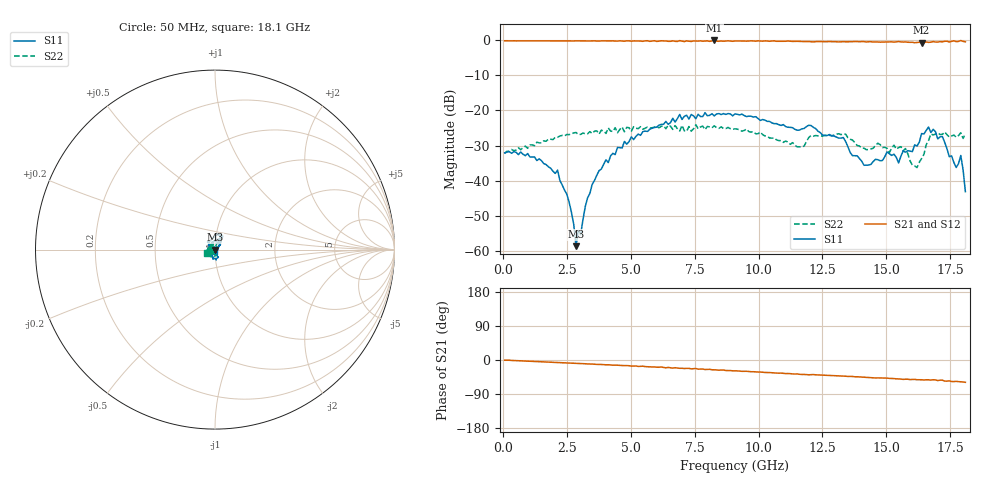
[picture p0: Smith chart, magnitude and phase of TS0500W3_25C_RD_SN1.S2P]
! Network Analyzer HP8720D.06.14 Serial No. US36140669
! 17 Jun 2005  06:18:02
! Frequency  S11  S21  S12  S22
# HZ  S  DB R 50
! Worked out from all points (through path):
!   201 points, 50 MHz to 18.1 GHz, reference 50 ohm
!   highest |S21| = -0.12 dB at 8.263 GHz (marker M1); lowest = -0.8 dB at 16.39 GHz (marker M2)
!   group delay of S21, straight-line fit = 8.93 ps
!   lowest |S11| = -58.6 dB at 2.848 GHz (marker M3), VSWR 1.00, Z = 50 - j0.116 ohm
!   |S11| at or under -10 dB: start of sweep to end of sweep
!   |S22| runs from -36.3 to -24.1 dB; largest |S21 - S12| = 0.032
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5e7  -32.05 -173.6  -0.21 -0.6  -0.22 -0.4  -32.23 -173.8
2.12575e9  -36.99 -158.3  -0.24 -6.7  -0.25 -6.6  -27.64 116.3
2.577e9  -46.07 -144.2  -0.25 -8.1  -0.26 -7.9  -26.88 108.3
2.84775e9  -58.59 -82.1  -0.24 -9.0  -0.26 -8.8  -26.28 103.4
3.1185e9  -51.11 -10.9  -0.25 -9.6  -0.29 -9.7  -26.45 98.5
3.4795e9  -41.05 22.2  -0.25 -10.7  -0.22 -10.7  -26.57 95.8
4.021e9  -34.03 33.4  -0.28 -12.7  -0.28 -12.3  -26.56 85.6
6.09675e9  -24.20 57.7  -0.32 -19.1  -0.24 -18.8  -24.94 68.0
8.26275e9  -21.58 74.3  -0.12 -26.0  -0.24 -26.5  -24.38 57.4
9.075e9  -21.00 79.8  -0.26 -28.5  -0.26 -28.4  -25.23 58.3
1.151175e10  -25.63 124.7  -0.36 -36.8  -0.32 -36.8  -30.37 83.1
1.21435e10  -24.82 131.2  -0.51 -38.5  -0.47 -38.5  -27.32 107.0
1.331675e10  -27.71 145.2  -0.46 -42.3  -0.49 -42.5  -26.69 102.8
1.4129e10  -35.60 179.7  -0.45 -45.3  -0.45 -45.3  -30.75 116.6
1.512175e10  -32.31 -122.1  -0.53 -48.5  -0.47 -48.0  -32.00 128.7
1.548275e10  -34.95 -101.6  -0.44 -49.9  -0.60 -49.8  -30.58 114.9
1.638525e10  -26.58 -68.1  -0.79 -52.1  -0.61 -51.9  -33.68 -64.2
1.674625e10  -26.27 -92.5  -0.60 -53.0  -0.72 -52.8  -26.67 -108.6
1.71975e10  -27.44 -109.8  -0.51 -53.3  -0.46 -51.9  -26.82 -130.8
1.7739e10  -36.23 -139.1  -0.46 -56.3  -0.58 -56.3  -27.62 -146.5
1.79195e10  -32.83 -171.4  -0.14 -57.6  -0.04 -56.1  -26.34 -158.8
1.81e10  -43.09 176.0  -0.51 -58.9  -0.46 -59.6  -26.61 -158.2
